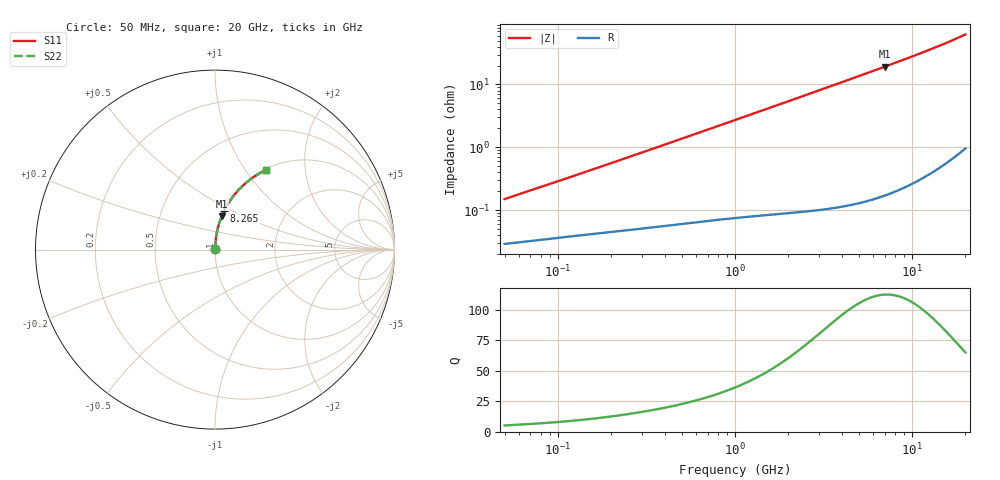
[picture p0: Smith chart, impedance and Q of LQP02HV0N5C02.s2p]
!Murata Part Number: LQP02HV0N5C02
!These Parameters are Measured in Series Mode Connection
!  o--[Z]--o
!Port1  Port2
!  o-------o
!Freq. Start=50[MHz] Stop=20[GHz], 401[Steps]
# Hz S RI R 50
!Freq.(Hz) S11(Real) S11(Imag) S21(Real) S21(Imag) S12(Real) S12(Imag) S22(Real) S22(Imag)
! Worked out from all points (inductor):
!   401 points, 50 MHz to 20 GHz, reference 50 ohm
!   read as one part in series: L = 463 pH near 51.52 MHz
!   highest Q = 113 at 7.009 GHz (marker M1), where L = 436 pH
!   S11 on the Smith chart (normalised r, x): 50 MHz: 1.00, +0.00; 8.265 GHz: 1.00, +0.46; 20 GHz: 1.02, +1.25
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5e7  0.000292 0.00147  0.9997 -0.00147  0.9997 -0.00147  0.000292 0.00147
5.152053e7  0.000295 0.00151  0.9997 -0.00151  0.9997 -0.00151  0.000295 0.00151
1.364002e8  0.000413 0.00385  0.9996 -0.00385  0.9996 -0.00385  0.000413 0.00385
3.721004e8  0.000652 0.0102  0.9993 -0.0102  0.9993 -0.0102  0.000652 0.0102
1e9  0.00148 0.0271  0.9985 -0.0271  0.9985 -0.0271  0.00148 0.0271
1.714689e9  0.003 0.0462  0.997 -0.0462  0.997 -0.0462  0.003 0.0462
2.728004e9  0.00636 0.0732  0.9936 -0.0732  0.9936 -0.0732  0.00636 0.0732
3.572216e9  0.0103 0.0955  0.9897 -0.0955  0.9897 -0.0955  0.0103 0.0955
4.539627e9  0.0161 0.121  0.9839 -0.121  0.9839 -0.121  0.0161 0.121
5.683258e9  0.0247 0.1507  0.9753 -0.1507  0.9753 -0.1507  0.0247 0.1507
7.009217e9  0.037 0.1845  0.963 -0.1845  0.963 -0.1845  0.037 0.1845
7.442007e9  0.0416 0.1953  0.9584 -0.1953  0.9584 -0.1953  0.0416 0.1953
8.264682e9  0.0511 0.2157  0.9489 -0.2157  0.9489 -0.2157  0.0511 0.2157
9.457416e9  0.0665 0.2446  0.9335 -0.2446  0.9335 -0.2446  0.0665 0.2446
1.066139e10  0.0841 0.2728  0.9159 -0.2728  0.9159 -0.2728  0.0841 0.2728
1.201863e10  0.1063 0.3032  0.8937 -0.3032  0.8937 -0.3032  0.1063 0.3032
1.334722e10  0.1305 0.3315  0.8695 -0.3315  0.8695 -0.3315  0.1305 0.3315
1.482269e10  0.1601 0.3609  0.8399 -0.3609  0.8399 -0.3609  0.1601 0.3609
1.621653e10  0.1905 0.3864  0.8095 -0.3864  0.8095 -0.3864  0.1905 0.3864
1.774144e10  0.2263 0.4117  0.7737 -0.4117  0.7737 -0.4117  0.2263 0.4117
1.940974e10  0.2684 0.4358  0.7316 -0.4358  0.7316 -0.4358  0.2684 0.4358
2e10  0.2839 0.4433  0.7161 -0.4433  0.7161 -0.4433  0.2839 0.4433
